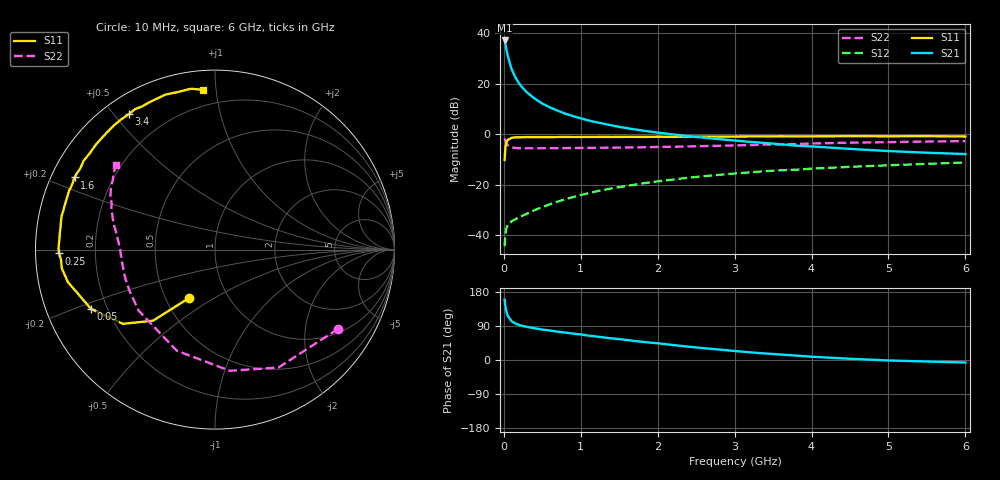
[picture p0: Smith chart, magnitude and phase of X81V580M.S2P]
! SIEMENS Small Signal Semiconductors
! BFP136W
! Si NPN RF Bipolar Junction Transistor in SOT343
! VCE = 1.5 V  IC = 80 mA
! Common Emitter S-Parameters:  September  1994
# GHz  S  MA  R  50
!  f  S11  S21  S12  S22
! GHz  MAG  ANG  MAG  ANG  MAG  ANG  MAG  ANG
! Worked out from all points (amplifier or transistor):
!   40 points, 10 MHz to 6 GHz, reference 50 ohm
!   highest |S21| = 37.1 dB at 10 MHz (marker M1)
!   |S21| within 3 dB of that: start of sweep to 30.01 MHz
!   unconditionally stable (mu >= 1): 486.8 MHz to 2.984 GHz
!   at 200 MHz: K = 0.68, MSG = 26.4 dB, |S12| = -32.9 dB
!   at 1.5 GHz: K = 1.12, MAG = 9.8 dB, |S12| = -21.0 dB
!   at 6 GHz: K = 0.99, MSG = 1.7 dB, |S12| = -11.3 dB
!   S11 on the Smith chart (normalised r, x): 10 MHz: 0.65, -0.39; 50 MHz: 0.14, -0.22; 250 MHz: 0.07, -0.01; 1.6 GHz: 0.07, +0.24; 3.4 GHz: 0.07, +0.55; 6 GHz: 0.10, +0.92
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0.01  0.3072 -118.3  71.44 159.2  0.006 69.3  0.8159 -32.8
0.02  0.5257 -131.1  60.64 142.3  0.0101 55.8  0.7461 -61.7
0.03  0.6588 -141.1  50.58 130.5  0.0131 47.5  0.6803 -83.0
0.05  0.7655 -154.4  35.63 116.6  0.0158 36.3  0.6023 -110.7
0.1  0.8397 -167.6  19.52 102.5  0.0186 33.7  0.5448 -141.3
0.15  0.8599 -173.1  13.25 96.3  0.0205 36.1  0.529 -153.8
0.2  0.8594 -176.0  9.929 92.5  0.0226 39.6  0.525 -160.4
0.25  0.869 -178.6  8.014 89.7  0.0243 43.3  0.5237 -164.6
0.3  0.8722 179.6  6.692 87.5  0.0264 46.3  0.522 -167.5
0.4  0.8689 176.2  5.042 83.6  0.031 50.5  0.5224 -171.3
0.5  0.8695 173.6  4.02 80.4  0.0358 54.3  0.5227 -173.9
0.6  0.8696 171.8  3.356 77.8  0.0406 56.3  0.524 -175.6
0.7  0.873 169.2  2.893 74.7  0.0459 58.7  0.5252 -176.9
0.9  0.8727 165.8  2.266 69.7  0.0562 60.0  0.5274 -179.4
1.1  0.8736 161.4  1.857 64.2  0.0672 60.7  0.5316 179.0
1.6  0.8801 152.8  1.308 52.9  0.0938 59.3  0.5416 175.0
2.2  0.8805 142.6  0.98 39.6  0.1256 54.9  0.5592 170.2
3.2  0.8942 125.7  0.699 20.3  0.1742 45.4  0.6043 161.2
3.4  0.8942 122.6  0.663 17.2  0.1839 43.2  0.6173 159.4
4.5  0.9065 107.8  0.508 3.2  0.224 32.9  0.6736 149.4
5.5  0.9065 98.6  0.426 -4.0  0.2567 24.9  0.7103 142.5
6  0.8931 94.3  0.401 -6.6  0.2732 20.5  0.724 139.5
